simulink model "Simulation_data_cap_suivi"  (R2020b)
settings: Solver=ode3  StartTime=0  StopTime=5  FixedStep=0.1  EnableMultiTasking=on
model workspace (MAT data in the model file):
  idcan = 1
libraries: fl_lib x3, nesl_utility x3, simulink_extras x1

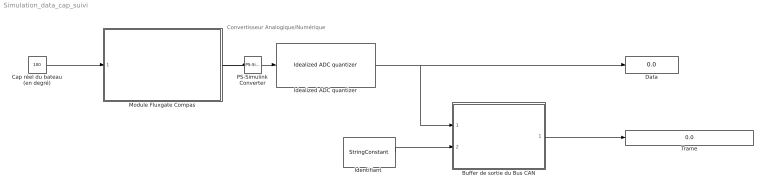
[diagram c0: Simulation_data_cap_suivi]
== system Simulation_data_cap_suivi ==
  note: Convertisseur Analogique/Numérique
  Buffer de sortie du Bus CAN : Subsystem
  Cap réel du bateau (en degré) : Constant  Value=100
  Data : Display
  Idealized ADC quantizer : simulink_extras/Additional Discrete/Idealized ADC quantizer  NumberOfConverterBits=10  Vmin=0  Vmax=5  OutputDataType=int16  OutputNegativeValues=off
  "Identifiant " : StringConstant  String="\"09F11200\""
  Module Fluxgate Compas : Subsystem
  PS-Simulink Converter : nesl_utility/PS-Simulink Converter  PhysicalDomain=network_engine_domain  SubClassName=ps_output  LeftPortType=input  RightPortType=output  PseudoPeriodic=off  Frequencies=[]  Unit=1  AffineConversion=off
  Trame : Display
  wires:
  PS-Simulink Converter/1 -> Idealized ADC quantizer/1
  Cap réel du bateau (en degré)/1 -> Module Fluxgate Compas/1(In1)
  "Identifiant "/1 -> Buffer de sortie du Bus CAN/2(In2)
  Buffer de sortie du Bus CAN/1(Out1) -> Trame/1
  Idealized ADC quantizer/1 -> Buffer de sortie du Bus CAN/1(u), Data/1
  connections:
  PS-Simulink Converter/LConn1 -- Module Fluxgate Compas/RConn1

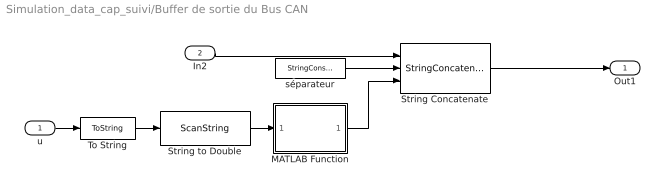
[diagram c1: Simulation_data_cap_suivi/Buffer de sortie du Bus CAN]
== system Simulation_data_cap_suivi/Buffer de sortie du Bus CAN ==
  u : Inport
  In2 : Inport  Port=2
  MATLAB Function : MATLAB Function  TreatAsAtomicUnit=on
  String Concatenate : StringConcatenate  Inputs=3
  String to Double : ScanString  Format="\"%lf\""
  To String : ToString
  séparateur : StringConstant  String="\" : \""
  Out1 : Outport
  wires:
  séparateur/1 -> String Concatenate/2
  String Concatenate/1 -> Out1/1
  In2/1 -> String Concatenate/1
  u/1 -> To String/1
  MATLAB Function/1(hexOut) -> String Concatenate/3
  To String/1 -> String to Double/1
  String to Double/1 -> MATLAB Function/1(data)

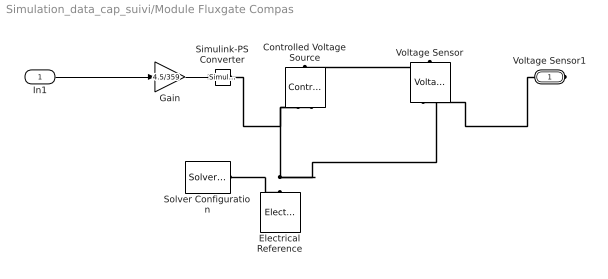
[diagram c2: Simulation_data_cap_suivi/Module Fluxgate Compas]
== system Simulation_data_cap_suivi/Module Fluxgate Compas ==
  In1 : Inport
  Controlled Voltage Source : fl_lib/Electrical/Electrical Sources/Controlled Voltage Source
  Electrical Reference : fl_lib/Electrical/Electrical Elements/Electrical Reference
  Gain : Gain  Gain=4.5/359
  Simulink-PS Converter : nesl_utility/Simulink-PS Converter  PhysicalDomain=network_engine_domain  SubClassName=ps_input  LeftPortType=input  RightPortType=output  PseudoPeriodic=off  Frequencies=[]  NoiseDistribution=none  NoiseParameters=[]  Unit=1  AffineConversion=off  FilteringAndDerivatives=provide  SimscapeFilterOrder=1  InputFilterTimeConstant=0.001  UdotUserProvided=0
  Solver Configuration : nesl_utility/Solver Configuration  PhysicalDomain=network_engine_domain  SubClassName=solver  LeftPortType=input  RightPortType=generic  Tones=[]  Harmonics=[]  SimulateNoise=off  Profile=off  UseLocalSampling=off  EnableSwitchedLinearOptims=on  FrequencyDomain=off  UseCCode=off  RelTol=0.001  AbsTol=1e-06  MinStep=1e-09  ToWorkspace=off  RevertToSquareIcSolve=off  NumHomotopyIterations=100  PhasorMode=off  PhasorModeNumHarmonics=1  DoDC=on  ResidualTolerance=0.1  UseLocalSolver=off  LocalSolverChoice=NE_BACKWARD_EULER_ADVANCER  LocalSolverSampleTime=.001  DoFixedCost=off  MaxNonlinIter=3  MaxModeIter=2  ComputeImpulses=off  ImpulseIterations=2  LinearAlgebra=Sparse  EquationFormulation=NE_TIME_EF  DelaysMemoryBudget=1024  AutomaticFiltering=on  FilteringTimeConstant=0.001  PartitionStorageMethod=AS_NEEDED  PartitionMemoryBudget=1024  PartitionMethod=FAST
  Voltage Sensor : fl_lib/Electrical/Electrical Sensors/Voltage Sensor
  Voltage Sensor1 : PMIOPort  Side=Right
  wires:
  Gain/1 -> Simulink-PS Converter/1
  In1/1 -> Gain/1
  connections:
  Solver Configuration/RConn1 -- Voltage Sensor/RConn2 -- Controlled Voltage Source/RConn2 -- Electrical Reference/LConn1
  Voltage Sensor/LConn1 -- Controlled Voltage Source/LConn1
  Voltage Sensor1/RConn1 -- Voltage Sensor/RConn1
  Simulink-PS Converter/RConn1 -- Controlled Voltage Source/RConn1

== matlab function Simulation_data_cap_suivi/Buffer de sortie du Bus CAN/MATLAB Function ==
function hexOut = conv(data)
    conv = dec2hex(data, 4);
    str2 = string(conv(3:4)); 
    str1 = string(conv(1:2)); 
    conv = "00 " + str2 + " " + str1 + " 00 00 00 00 00";
    hexOut=conv;
  
    
end
